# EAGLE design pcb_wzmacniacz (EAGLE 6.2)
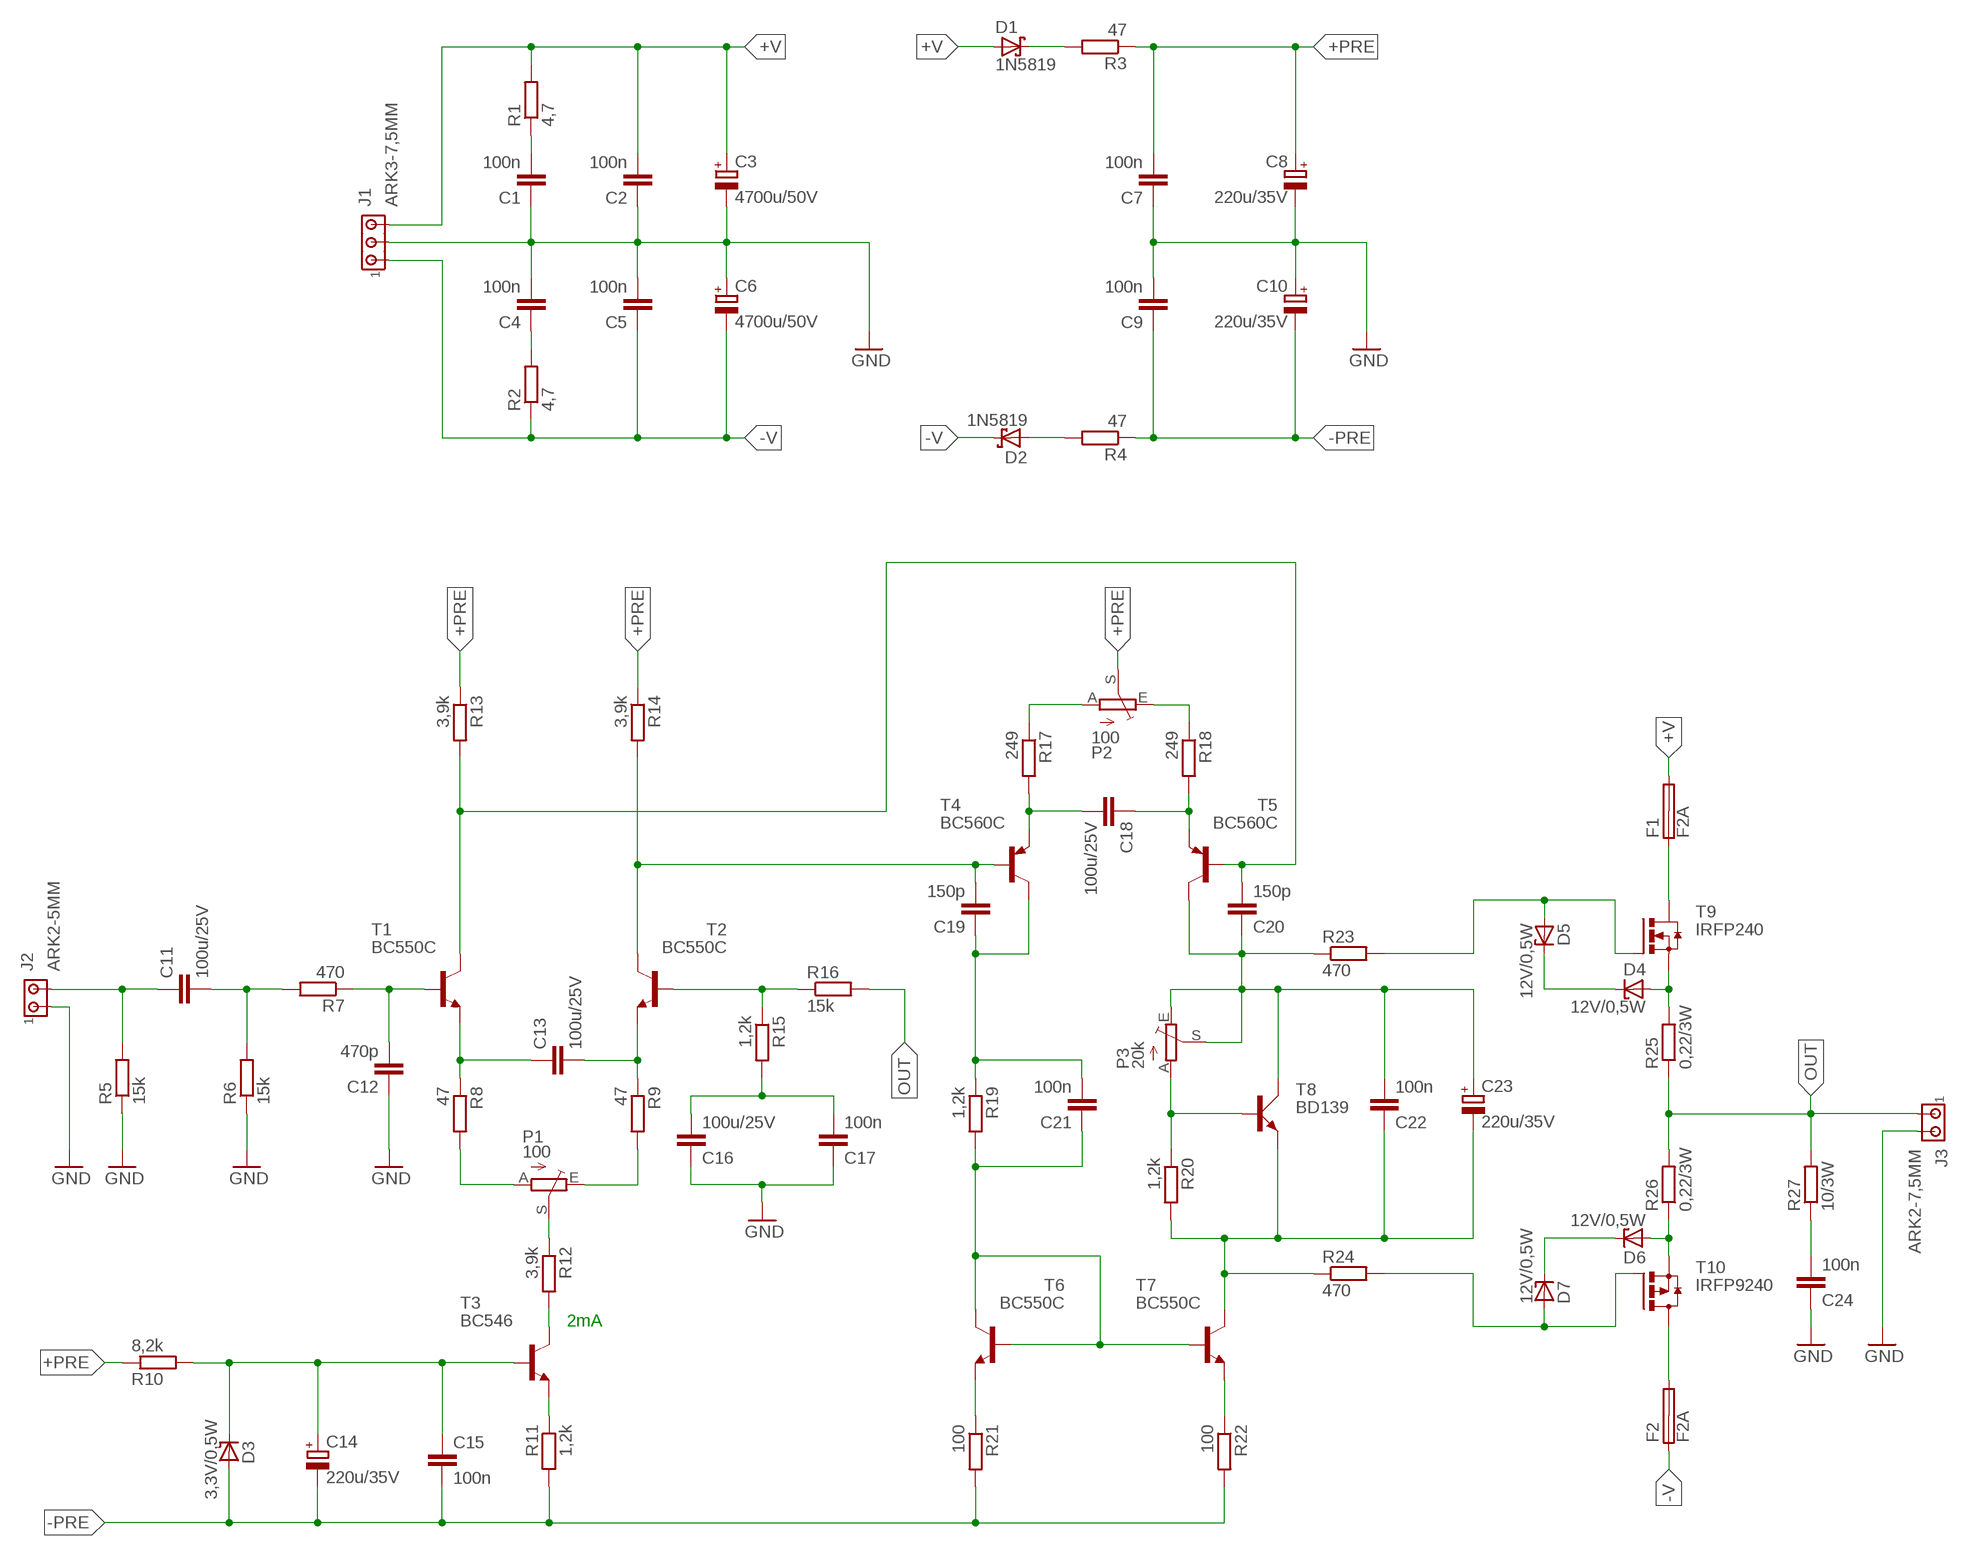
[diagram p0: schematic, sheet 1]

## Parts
C1  100n  C-EU050-025X075  [C050-025X075]
C2  100n  C-EU050-025X075  [C050-025X075]
C3  4700u/50V  CPOL-EUE10-22.5  [EB22,5D]
C4  100n  C-EU050-025X075  [C050-025X075]
C5  100n  C-EU050-025X075  [C050-025X075]
C6  4700u/50V  CPOL-EUE10-22.5  [EB22,5D]
C7  100n  C-EU050-025X075  [C050-025X075]
C8  220u/35V  CPOL-EUE3.5-8  [E3,5-8]
C9  100n  C-EU050-025X075  [C050-025X075]
C10  220u/35V  CPOL-EUE3.5-8  [E3,5-8]
C11  100u/25V  C-EU050-075X075  [C050-075X075]
C12  470p  C-EU050-025X075  [C050-025X075]
C13  100u/25V  C-EU050-075X075  [C050-075X075]
C14  220u/35V  CPOL-EUE3.5-8  [E3,5-8]
C15  100n  C-EU050-025X075  [C050-025X075]
C16  100u/25V  C-EU050-075X075  [C050-075X075]
C17  100n  C-EU050-025X075  [C050-025X075]
C18  100u/25V  C-EU050-075X075  [C050-075X075]
C19  150p  C-EU050-025X075  [C050-025X075]
C20  150p  C-EU050-025X075  [C050-025X075]
C21  100n  C-EU050-025X075  [C050-025X075]
C22  100n  C-EU050-025X075  [C050-025X075]
C23  220u/35V  CPOL-EUE3.5-8  [E3,5-8]
C24  100n  C-EU050-025X075  [C050-025X075]
D1  1N5819  1N5819-B  [DO41-7.6]
D2  1N5819  1N5819-B  [DO41-7.6]
D3  3,3V/0,5W  ZENER-DIODEDO34-7  [DO34Z7]
D4  12V/0,5W  ZENER-DIODEDO34-7  [DO34Z7]
D5  12V/0,5W  ZENER-DIODEDO34-7  [DO34Z7]
D6  12V/0,5W  ZENER-DIODEDO34-7  [DO34Z7]
D7  12V/0,5W  ZENER-DIODEDO34-7  [DO34Z7]
F1  F2A  SHK20L  [SHK20L]
F2  F2A  SHK20L  [SHK20L]
J1  ARK3-7,5MM  [3PIN-7,5MM]
J2  ARK2-5MM  [2PIN-5MM]
J3  ARK2-7,5MM  [2PIN-7,5MM]
P1  100  TRIM_EU-CA6V  [CA6V]
P2  100  TRIM_EU-CA6V  [CA6V]
P3  20k  TRIM_EU-B64Y  [B64Y]
R1  4,7  R-EU_0207/12  [0207/12]
R2  4,7  R-EU_0207/12  [0207/12]
R3  47  R-EU_0207/7  [0207/7]
R4  47  R-EU_0207/7  [0207/7]
R5  15k  R-EU_0207/7  [0207/7]
R6  15k  R-EU_0207/7  [0207/7]
R7  470  R-EU_0207/7  [0207/7]
R8  47  R-EU_0207/7  [0207/7]
R9  47  R-EU_0207/7  [0207/7]
R10  8,2k  R-EU_0207/7  [0207/7]
R11  1,2k  R-EU_0207/7  [0207/7]
R12  3,9k  R-EU_0207/7  [0207/7]
R13  3,9k  R-EU_0207/7  [0207/7]
R14  3,9k  R-EU_0207/7  [0207/7]
R15  1,2k  R-EU_0207/7  [0207/7]
R16  15k  R-EU_0207/7  [0207/7]
R17  249  R-EU_0207/7  [0207/7]
R18  249  R-EU_0207/7  [0207/7]
R19  1,2k  R-EU_0207/7  [0207/7]
R20  1,2k  R-EU_0207/7  [0207/7]
R21  100  R-EU_0207/7  [0207/7]
R22  100  R-EU_0207/7  [0207/7]
R23  470  R-EU_0207/7  [0207/7]
R24  470  R-EU_0207/7  [0207/7]
R25  0,22/3W  R-EU_0617/17  [0617/17]
R26  0,22/3W  R-EU_0617/17  [0617/17]
R27  10/3W  R-EU_0617/17  [0617/17]
T1  BC550C  BC546B  [TO92-EBC]
T2  BC550C  BC546B  [TO92-EBC]
T3  BC546  BC546B  [TO92-EBC]
T4  BC560C  [TO92-EBC]
T5  BC560C  [TO92-EBC]
T6  BC550C  BC546B  [TO92-EBC]
T7  BC550C  BC546B  [TO92-EBC]
T8  BD139  [TO126AV]
T9  IRFP240  [TO247BV]
T10  IRFP9240  [TO247BV]

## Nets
+PRE: C7.2 C8.+ P2.S R3.1 R10.1 R13.1 R14.1
+V: C2.2 C3.+ D1.A F1.2A J1.P3 R1.2
-PRE: C9.1 C10.- C14.- C15.2 D3.A R4.1 R11.2 R21.2 R22.2
-V: C5.1 C6.- D2.C F2.1A J1.P1 R2.1
GND: C1.1 C2.1 C3.- C4.2 C5.2 C6.+ C7.1 C8.- C9.2 C10.+ C12.1 C16.1 C17.1 C24.1 J1.P2 J2.P$1 J3.P2 R5.1 R6.1
N$1: P1.A R8.2
N$2: C11.1 J2.P$2 R5.2
N$3: D1.C R3.2
N$4: P1.E R9.2
N$5: P2.A R17.1
N$6: P2.E R18.1
N$7: C11.2 R6.2 R7.2
N$8: C12.2 R7.1 T1.B
N$9: D2.A R4.2
N$10: C1.2 R1.1
N$11: P3.A R20.1 T8.B
N$12: C22.1 C23.- R20.2 R24.1 T7.C T8.E
N$13: C20.1 C22.2 C23.+ P3.E P3.S R23.1 T5.C T8.C
N$14: D4.C D5.C
N$15: D5.A R23.2 T9.G
N$16: D6.A R26.1 T10.S
N$18: D4.A R25.2 T9.S
N$19: D6.C D7.C
N$20: D7.A R24.2 T10.G
N$21: F1.1A T9.D
N$22: C24.2 R27.1
N$23: C4.1 R2.2
N$24: C13.1 R8.1 T1.E
N$25: C13.2 R9.1 T2.E
N$26: P1.S R12.1
N$27: R12.2 T3.C
N$28: C14.+ C15.1 D3.C R10.2 T3.B
N$29: R11.1 T3.E
N$30: C16.2 C17.2 R15.2
N$31: R15.1 R16.1 T2.B
N$32: C20.2 R13.2 T1.C T5.B
N$33: C19.2 R14.2 T2.C T4.B
N$34: C18.2 R17.2 T4.E
N$35: C18.1 R18.2 T5.E
N$36: C19.1 C21.2 R19.1 T4.C
N$37: F2.2A T10.D
N$38: C21.1 R19.2 T6.B T6.C T7.B
N$39: R21.1 T6.E
N$40: R22.1 T7.E
OUT: J3.P1 R16.2 R25.1 R26.2 R27.2
Unconnected: F1.1B F1.2B F2.1B F2.2B

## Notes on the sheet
- 2mA

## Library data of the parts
C1 C2 C4 C5 C7 C9 C11-C13 C15-C22 C24 = rcl:C-EU: CAPACITOR, European symbol
C3 C6 C8 C10 C14 C23 = rcl:CPOL-EU: POLARIZED CAPACITOR, European symbol
D1 D2 = diode:1N581*: 1.0A SCHOTTKY BARRIER RECTIFIER
D3-D7 = diode:ZENER-DIODE: Z-Diode
F1 F2 = fuse:SHK20L: FUSE HOLDER 5 x 20 mm, SH contact, SHH1 Schukat, E1073 Buerklin; OC_FARNELL: unknown; OC_NEWARK: unknown
J1 = zlacza_futrzak:ARK3: ARK 3 Raster 5mm i 3,5mm
J2 J3 = zlacza_futrzak:ARK2: ARK 2
P1-P3 = pot:TRIM_EU-: POTENTIOMETER
R1-R27 = rcl:R-EU_: RESISTOR, European symbol
T1-T3 T6 T7 = transistor-npn:BC546*: NPN Transistor
T4 T5 = transistor-pnp:BC560*: PNP Transistror
T8 = transistor-power:BD139: NPN TRANSISTOR
T9 = transistor-power:IRFP240: HEXFET Power MosFet Source: http://www.irf.com/
T10 = inne_futrzak:IRFP9240

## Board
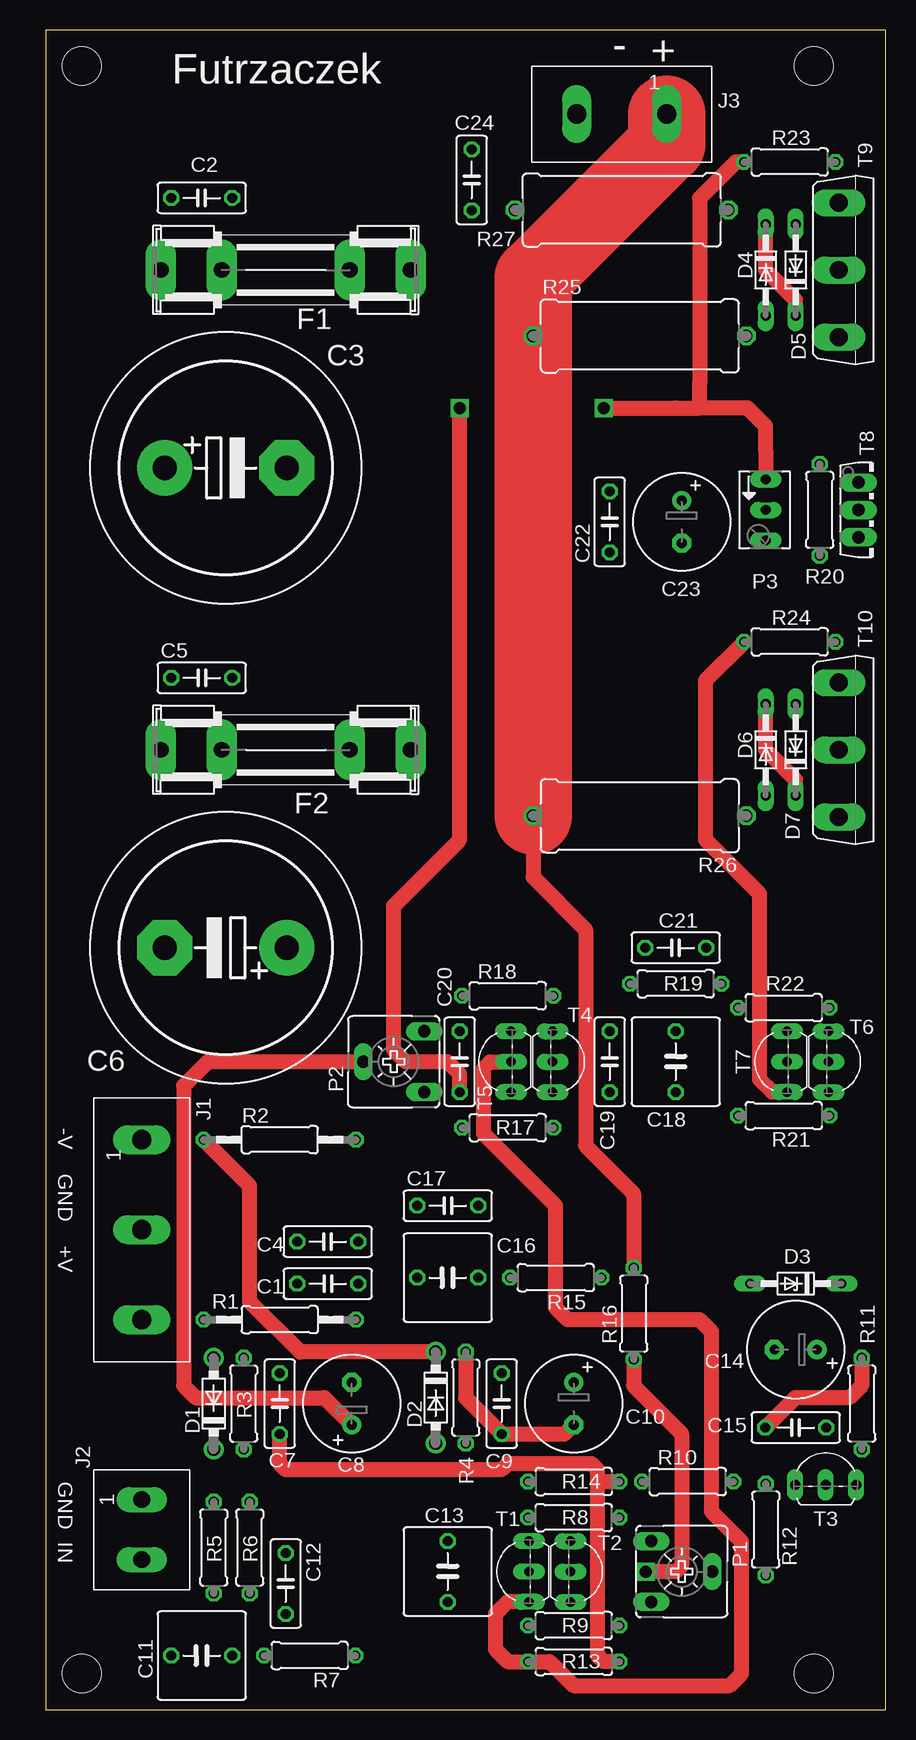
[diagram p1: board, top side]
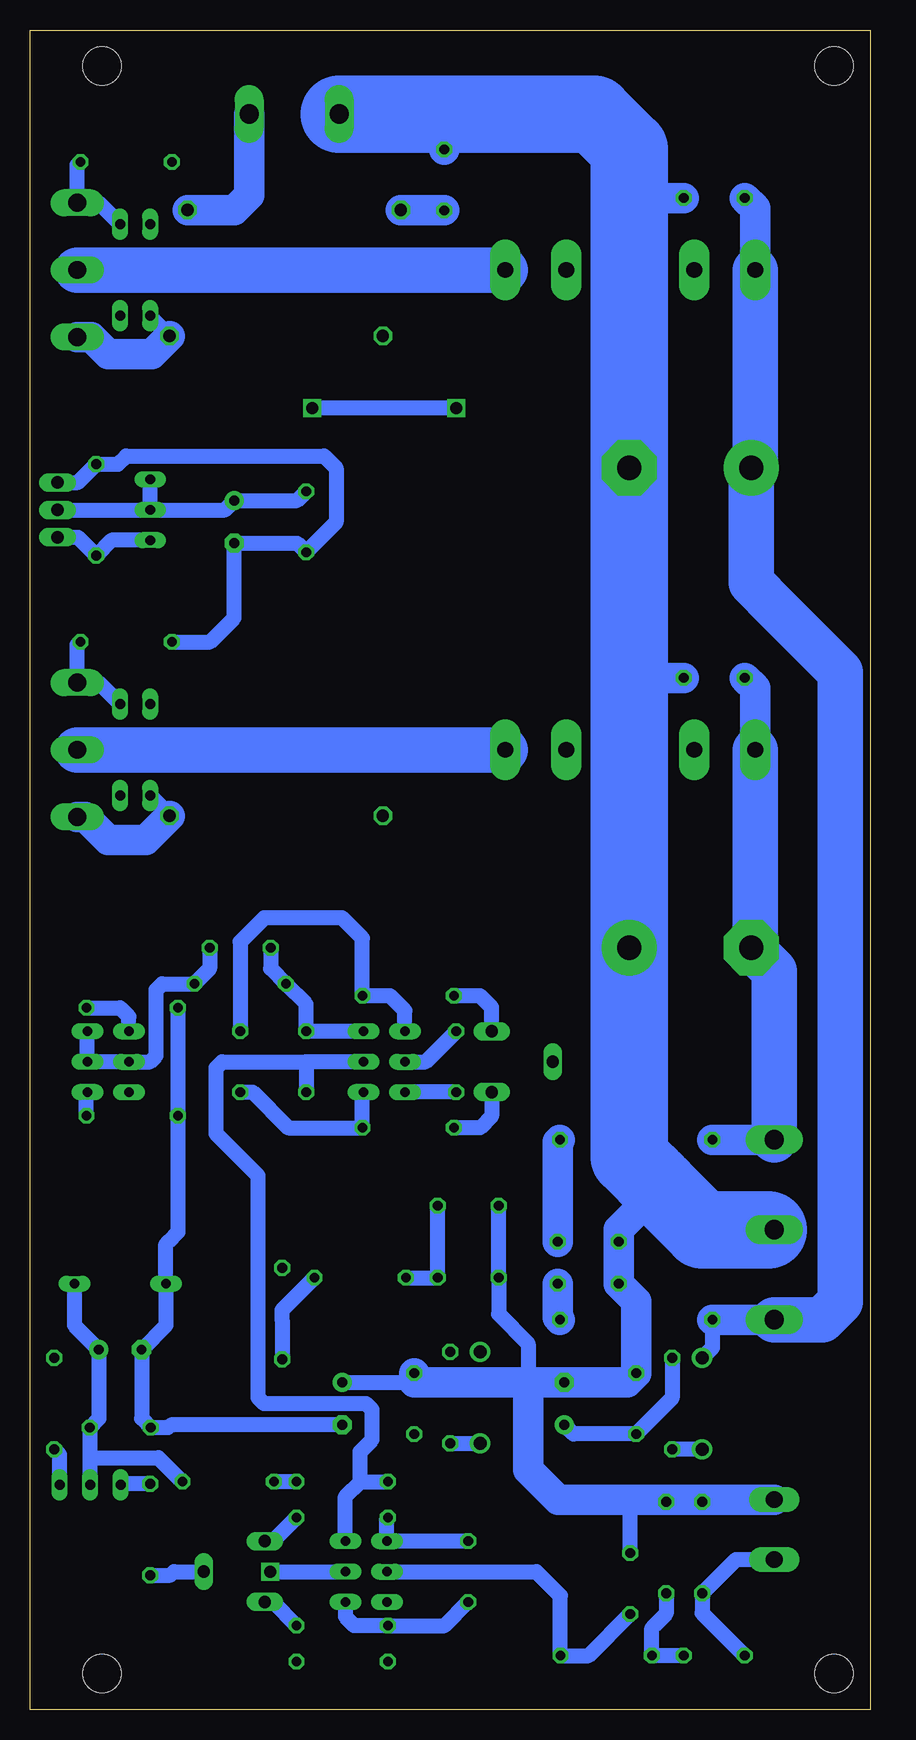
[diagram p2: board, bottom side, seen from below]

Size 70 x 140 mm. Coordinates in mm from the lower left corner, seen from the top.
Outline: 0,0 70,0 70,140 0,140 0,0
Copper layers (1*16): Top 0.035mm / dielectric 1.5mm / Bottom 0.035mm
Design rules: minimum track width 10mil, minimum drill 23mil, track to track 8mil, track to pad 8mil, pad to pad 8mil, via to via 8mil, smd to smd 8mil, copper to edge 20mil, drill to drill 8mil, minimum pad ring 10mil, minimum via ring 8mil, stop-mask expansion 4mil, vias tented up to drill 0mil, thermal gap 10mil
Holes 3.2 mm at 3,3 64,3 3,137 64,137

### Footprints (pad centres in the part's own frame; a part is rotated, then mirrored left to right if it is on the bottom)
C050-025X075 = drill 0.813 octagon: 1 -2.54,0; 2 2.54,0
EB22,5D = drill 2.007 pad 4.597: + -5.08,0 | drill 2.007 pad 4.597 octagon: - 5.08,0
E3,5-8 = drill 0.813 pad 1.6: + -1.778,0 | drill 0.813 pad 1.6 octagon: - 1.778,0
C050-075X075 = drill 0.813 octagon: 1 -2.54,0; 2 2.54,0
DO41-7.6 = drill 1.1 pad 1.7: A 3.81,0; C -3.81,0
DO34Z7 = drill 0.813 long: A 3.81,0; C -3.81,0
SHK20L = drill 1.321 pad 2.54 long: 1A -10.414,0; 1B -5.334,0; 2A 10.414,0; 2B 5.334,0
3PIN-7,5MM = drill 1.6 long: P1 -7.5,0; P2 0,0; P3 7.5,0
2PIN-5MM = drill 1.4 long: P$1 -2.5,0; P$2 2.5,0
2PIN-7,5MM = drill 1.6 long: P1 -3.75,0; P2 3.75,0
CA6V = drill 1.016 long: A -2.54,-2.54; E 2.54,-2.54; S 0,2.54
B64Y = drill 0.813 long: A 2.54,0; E -2.54,0; S 0,0
0207/12 = drill 0.813 octagon: 1 -6.35,0; 2 6.35,0
0207/7 = drill 0.813 octagon: 1 -3.81,0; 2 3.81,0
0617/17 = drill 1.016 octagon: 1 -8.89,0; 2 8.89,0
TO92-EBC = drill 0.813 long: B 0,-1.27; C -2.54,-1.27; E 2.54,-1.27
TO126AV = drill 1.016 long: B 2.286,-1.27; C 0,-1.27; E -2.286,-1.27
TO247BV = drill 1.499 long: D 0,-2.921; G -5.588,-2.921; S 5.588,-2.921

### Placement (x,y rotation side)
C1  23.5,35.5 0 top
C2  13,126 180 top
C3  15,103.5 0 top
C4  23.5,39 180 top
C5  13,86 0 top
C6  15,63.5 180 top
C7  19.5,25.5 270 top
C8  25.5,25.5 90 top
C9  38,25.5 90 top
C10  44,25.5 270 top
C11  13,4.5 0 top
C12  20,10.5 270 top
C13  33.5,11.5 270 top
C14  62.5,30 180 top
C15  62.5,23.5 180 top
C16  33.5,36 0 top
C17  33.5,42 0 top
C18  52.5,54 270 top
C19  47,54 270 top
C20  34.5,54 90 top
C21  52.5,63.5 180 top
C22  47,99 90 top
C23  53,99 270 top
C24  35.5,127.5 270 top
D1  14,25.5 90 top
D2  32.5,26 270 top
D3  62.5,35.5 180 top
D4  60,120 270 top
D5  62.5,120 90 top
D6  60,80 270 top
D7  62.5,80 90 top
F1  20,120 180 top
F2  20,80 0 top
J1  8,40 270 top
J2  8,15 270 top
J3  48,133 180 top
P1  53,11.5 270 top
P2  29,54 90 top
P3  60,100 270 top
R1  19.5,32.5 180 top
R2  19.5,47.5 0 top
R3  16.5,25.5 270 top
R4  35,26 270 top
R5  14,13.5 270 top
R6  17,13.5 270 top
R7  22,4.5 180 top
R8  44,16 0 top
R9  44,7 0 top
R10  53.5,19 0 top
R11  68,25.5 90 top
R12  60,15 90 top
R13  44,4 180 top
R14  44,19 180 top
R15  42.5,36 180 top
R16  49,33 90 top
R17  38.5,48.5 0 top
R18  38.5,59.5 0 top
R19  52.5,60.5 0 top
R20  64.5,100 90 top
R21  61.5,49.5 180 top
R22  61.5,58.5 180 top
R23  62,129 0 top
R24  62,89 0 top
R25  49.5,114.5 0 top
R26  49.5,74.5 180 top
R27  48,125 0 top
T1  39,11.5 90 top
T2  45,11.5 270 top
T3  65,20 0 top
T4  43.5,54 270 top
T5  37.5,54 90 top
T6  66.5,54 270 top
T7  60.5,54 90 top
T8  69,100 270 top
T9  69,120 270 top
T10  69,80 270 top

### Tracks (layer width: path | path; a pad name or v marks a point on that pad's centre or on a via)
+PRE
  Top 1.27: R13.1 46.5,4 46,4.5 46,19 | 46,19 46,20 45.5,20.5 39,20.5 38.5,20.5 38,20 20,20 19.5,20.5 C7.2 | R14.1 46,19 | P2.S 13.5,54 11.5,52 11.5,27 12.5,26 23.22,26 C8.+
  Bottom 1.27: R3.1 16.5,25.96 C7.2 24.74,22.96 C8.+ | R14.1 R10.1
+V
  Bottom 1.27: R1.2 13.15,30.16 D1.A
  Bottom 2.54: R1.2 J1.P3 | F1.2A 9.59,125.13 C2.2
  Bottom 3.81: J1.P3 4,32.5 2.5,34 2.5,86.5 7.75,91.75 | 7.75,91.75 8.5,92.5 | 7.75,91.75 9.92,93.92 C3.+ 9.59,103.83 F1.2A
-PRE
  Top 1.27: R4.1 35,25.96 C9.1 43.24,22.96 C10.- | R11.2 68,27 67,26 62.46,26 C15.2
  Bottom 1.27: C10.- 58.28,23.72 58.5,23.5 C15.2 60.72,24.26 C14.- 58.69,32.03 D3.A 58.69,38.81 58.5,39 57.69,39.81 R21.2 R22.2
-V
  Top 1.27: D2.C 21.19,29.81 17,34 17,43.65 R2.1
  Bottom 2.54: R2.1 J1.P1 | F2.1A 9.59,85.13 C5.1
  Bottom 3.81: F2.1A 9.59,63.5 C6.- 8,61.58 J1.P1
GND
  Bottom 1.27: R5.1 14,17.5 | R6.1 16.69,17.31 16.5,17.5 | C12.1 20,17.5 | 28.5,27.28 28.5,30.5 30.96,32.96 C16.1 C17.1 | C10.+ 38.22,27.28 38,27.5
  Bottom 2.54: C24.1 35.5,133 | 8.5,40 J1.P2 | 17.5,43.5 20.96,40.04 C4.2 C1.1 19.5,34.04 C7.1 20.26,27.28 C8.- 28.5,27.28 | C5.2 20.08,86 | C2.1 20.08,126 | 28.5,27.28 38,27.28 38,27.5 C9.2 | J2.P$1 14,17.5 16.5,17.5 20,17.5 26,17.5 28.5,20 28.5,27.28
  Bottom 6.452: 18,44 17.5,43.5 14,40 8.5,40 | 18,44 18.5,44.5 | 18,44 20.08,46.08 C6.+ 20.08,86 C3.- 20.08,126 20.08,130.08 23,133 35.5,133 J3.P2
N$1
  Bottom 1.27: P1.A 49.77,14.04 R8.2
N$2
  Bottom 1.27: J2.P$2 11.19,12.5 R5.2 14,8.04 C11.1
N$3
  Bottom 1.27: D1.C R3.2
N$4
  Bottom 1.27: P1.E 49.77,8.96 R9.2
N$5
  Bottom 1.27: P2.A 31.54,49.46 32.5,48.5 R17.1
N$6
  Bottom 1.27: P2.E 31.54,58.54 32.5,59.5 R18.1
N$7
  Bottom 1.27: C11.2 R7.2 18.19,6.81 18,7 17,8 R6.2
N$8
  Bottom 1.27: T1.B 27.81,11.5 25.81,9.5 R7.1 23.46,4.5 C12.2
N$9
  Bottom 1.27: R4.2 D2.A
N$10
  Bottom 2.54: C1.2 26.04,32.69 R1.1
N$11
  Bottom 1.27: T8.B 66.02,97.71 R20.1 63.23,97.46 P3.A
N$12
  Top 1.27: T7.C 60.54,51.46 59.5,52.5 59.5,68 56,71.5 55,72.5 55,85.81 R24.1
  Bottom 1.27: R24.1 55,89 53,91 C23.- 47.76,97.22 C22.1 44.5,98.96 44.5,103.5 45.5,104.5 62,104.5 62.69,103.81 R20.2 66.02,102.29 T8.E
N$13  (via drill 1)
  Top 1.27: R23.1 57.5,129 54.5,126 54.5,110.5 54.5,108.5 | P3.E 60,105 60,107 58.5,108.5 54.5,108.5 | C20.1 34.5,53 33.5,54 30,54 29,55 29,67 34.5,72.5 v34.5,108.5 | v46.5,108.5 52.5,108.5 54.5,108.5
  Bottom 1.27: C22.2 47.76,100.78 C23.+ 53.78,100 P3.S | T8.C P3.S | P3.S P3.E | v34.5,108.5 v46.5,108.5 | C20.1 T5.C
N$14
  Top 1.27: D5.C 62.5,117.5 60,120 D4.C
N$15
  Bottom 1.27: D5.A 64.28,125.59 T9.G 66.08,128.73 R23.2
N$16
  Bottom 1.27: R26.1 58.39,74.58 D6.A
  Bottom 2.54: T10.S 65.41,74.41 63.5,72.5 60.39,72.5 R26.1
N$18
  Bottom 1.27: D4.A 60,116.11 R25.2
  Bottom 2.54: R25.2 59.89,113 63.5,113 64.91,114.41 T9.S
N$19
  Top 1.27: D7.C 62.5,77.5 60,80 D6.C
N$20
  Bottom 1.27: D7.A 64.28,85.59 T10.G 66.08,88.73 R24.2
N$21
  Bottom 3.81: T9.D F1.1A
N$22
  Bottom 2.54: C24.2 35.54,125 R27.1
N$23
  Bottom 2.54: C4.1 26.04,47.31 R2.2
N$24
  Bottom 1.27: C13.1 T1.E 40.27,15.92 R8.1
N$25
  Bottom 1.27: T2.E 43.73,7.73 43.5,7.5 43,7 R9.1 35.46,7 C13.2
N$26
  Bottom 1.27: R12.1 58.31,11.19 58,11.5 P1.S
N$27
  Bottom 1.27: R12.2 62.38,18.81 T3.C
N$28
  Bottom 1.27: T3.B 65,21 | 65,21 59.31,21 R10.2 | 65,21 65,23.46 C15.1 64.28,24.26 C14.+ 66.31,32.03 D3.C
N$29
  Bottom 1.27: T3.E 67.54,21.23 R11.1
N$30
  Bottom 1.27: R15.2 C16.2 C17.2
N$31  (via drill 1)
  Top 1.27: R16.1 49,27 52.5,23.5 53,23 53,12 52.5,11.5 v50,11.5
  Bottom 1.27: R16.1 49,32.5 49,33.31 R15.1 | v50,11.5 T2.B
N$32
  Top 1.27: T1.C 38.46,8.96 38,8.5 37.5,8 37.5,5 38.5,4 R13.2 42,4 44,2 57,2 58,3 58,14 55.5,16.5 55.5,31.5 54.5,32.5 43.5,32.5 42.5,33.5 42.5,42 37,47.5 36.5,48 36.5,53.46 37.04,54 T5.B
  Bottom 1.27: T5.B 37.04,54 C20.2
N$33
  Bottom 1.27: T2.C 43.73,17.77 42.5,19 | 42.5,19 R14.2 | T4.B 47,54 | 47,54 C19.2 | 42.5,19 42.5,21.5 41.5,22.5 41.5,25 42,25.5 50.5,25.5 51,26 51,44.5 54.5,48 54.5,53.5 54,54 47,54
N$34
  Bottom 1.27: C18.2 51.46,51.46 48.5,48.5 R17.2 42.31,51.38 T4.E
N$35
  Bottom 1.27: T5.E 38.77,58.27 40,59.5 R18.2 42.31,64.31 44,66 50.5,66 52.5,64 C18.1
N$36
  Bottom 1.27: C21.2 49.96,61.77 R19.1 47,58.81 C19.1 T4.C
N$37
  Bottom 3.81: T10.D F2.2A
N$38
  Bottom 1.27: T6.C T6.B T7.B 60,54 59.5,54.5 59.5,60 59,60.5 R19.2 55.04,61.77 C21.1
N$39
  Bottom 1.27: R21.1 65.31,51.38 T6.E
N$40
  Bottom 1.27: R22.1 62.5,58.5 62,58 61.77,57.77 T7.E
OUT
  Top 1.27: R26.2 40.61,69.39 45,65 45,47 49,43 R16.2
  Top 6.452: R26.2 R25.1 40.61,119.36 51.75,130.5 51.75,131.5 | 51.75,130.64 51.75,131.5 | 51.75,131.5 J3.P1
  Bottom 2.54: R27.2 53,125 51.75,126.25 J3.P1

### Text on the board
tPlace: + - | Futrzaczek | -V GND +V | GND IN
